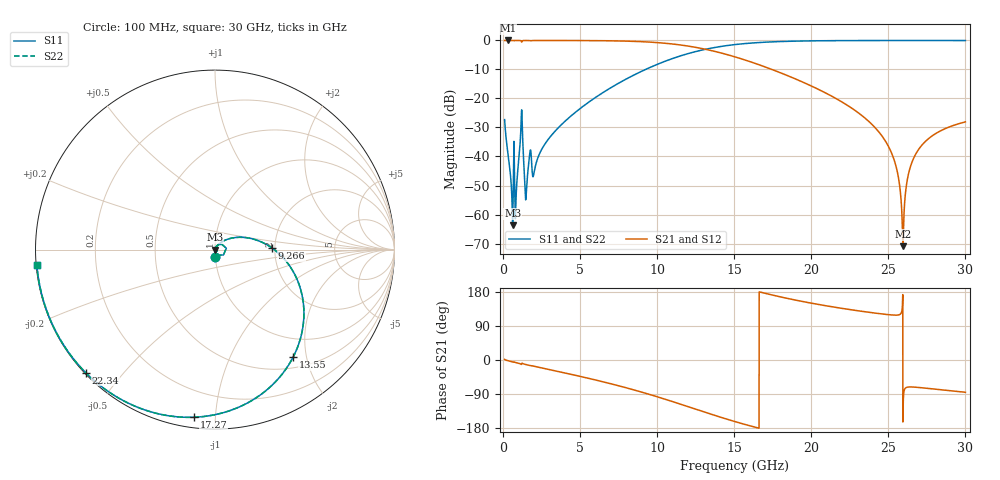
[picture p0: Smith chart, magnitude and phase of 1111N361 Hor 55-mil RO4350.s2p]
# GHz S MA R 50
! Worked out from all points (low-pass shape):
!   3201 points, 100 MHz to 30 GHz, reference 50 ohm
!   highest |S21| = 0.00 dB at 324.2 MHz (marker M1); lowest = -70.9 dB at 25.94 GHz (marker M2)
!   |S21| within 3 dB of the highest: start of sweep to 13.1 GHz
!   lowest |S11| = -63.7 dB at 623.2 MHz (marker M3), VSWR 1.00, Z = 50.1 - j0.000937 ohm
!   |S11| at or under -10 dB: start of sweep to 9.244 GHz
!   |S22| runs from -63.7 to 0.0 dB; largest |S21 - S12| = 0
!   S11 on the Smith chart (normalised r, x): 100 MHz: 1.00, -0.09; 9.266 GHz: 1.93, +0.04; 13.55 GHz: 0.67, -1.77; 17.27 GHz: 0.05, -0.88; 22.34 GHz: 0.00, -0.40; 30 GHz: 0.00, -0.04
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0.1  0.04319 -88.0  0.9988 1.7  0.9988 1.7  0.04319 -88.0
0.32425  0.01083 -90.1  0.9995 -2.0  0.9995 -2.0  0.01083 -90.1
0.62325  0.0006567 -0.8  0.9993 -5.0  0.9993 -5.0  0.0006567 -0.8
0.9035625  0.003887 70.6  0.9991 -7.5  0.9991 -7.5  0.003887 70.6
1.165188  0.03461 53.1  0.9844 -11.2  0.9844 -11.2  0.03461 53.1
1.501562  0.002249 28.2  0.9981 -12.2  0.9981 -12.2  0.002249 28.2
1.725812  0.0109 44.3  0.9941 -14.5  0.9941 -14.5  0.0109 44.3
2.024812  0.005518 50.2  0.9976 -16.6  0.9976 -16.6  0.005518 50.2
5.089563  0.06991 44.9  0.9956 -44.0  0.9956 -44.0  0.06991 44.9
9.266219  0.3182 1.6  0.9445 -88.0  0.9445 -88.0  0.3182 1.6
10.06978  0.3935 -8.2  0.9154 -97.8  0.9154 -97.8  0.3935 -8.2
13.54566  0.7405 -54.0  0.6661 -143.7  0.6661 -143.7  0.7405 -54.0
15.05  0.8491 -72.9  0.521 -162.6  0.521 -162.6  0.8491 -72.9
17.27381  0.9409 -97.0  0.3289 173.3  0.3289 173.3  0.9409 -97.0
20.03956  0.9838 -120.7  0.1624 149.7  0.1624 149.7  0.9838 -120.7
22.33813  0.9944 -136.4  0.07636 134.1  0.07636 134.1  0.9944 -136.4
25.01978  0.9973 -151.8  0.01471 119.6  0.01471 119.6  0.9973 -151.8
25.57106  0.9974 -154.6  0.005645 118.5  0.005645 118.5  0.9974 -154.6
25.94481  0.9974 -156.5  0.0002847 -163.6  0.0002847 -163.6  0.9974 -156.5
26.33725  0.9973 -158.5  0.005413 -71.2  0.005413 -71.2  0.9973 -158.5
26.94459  0.9973 -161.4  0.01302 -72.4  0.01302 -72.4  0.9973 -161.4
30  0.9965 -175.1  0.03948 -85.2  0.03948 -85.2  0.9965 -175.1
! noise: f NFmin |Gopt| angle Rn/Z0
0.1  0.0006726  0.7368  0.9267  0.0005108
3.417  0.008899  0.4458  26.71  0.002551
6.743  0.01533  0.4111  48.66  0.003637
10.06  0.02395  0.4614  66.59  0.005534
13.39  0.03817  0.5723  83.95  0.009464
16.7  0.06703  0.7194  103.3  0.01898
20.03  0.1421  0.8566  123.8  0.04795
23.35  0.4558  0.9526  143  0.2188
26.67  2.32  0.99  160.1  1.667
30  0.6059  0.9611  175  0.008058
